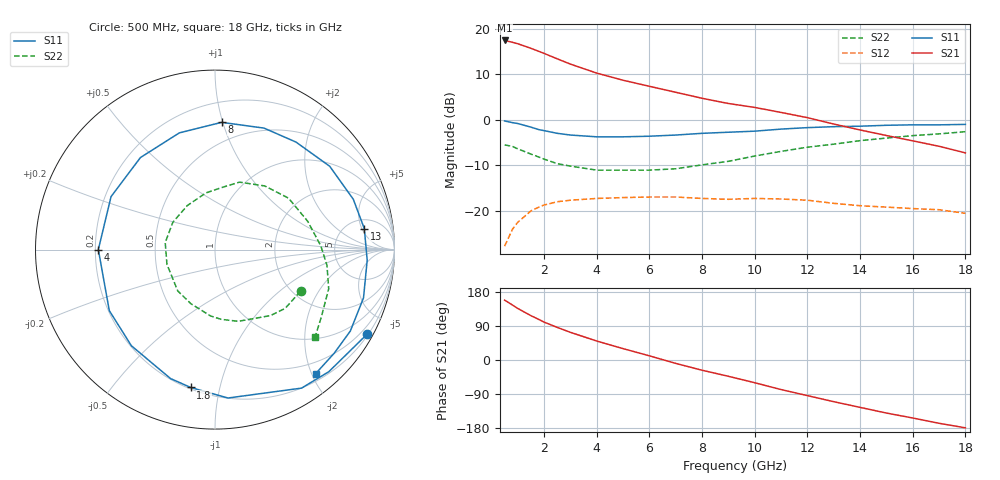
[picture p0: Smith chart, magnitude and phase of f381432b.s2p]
!ATF-38143
!S-PARAMETERS at Vds=2V  Id=10mA.  LAST UPDATED 20-10-99
# ghz s ma r 50
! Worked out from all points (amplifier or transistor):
!   23 points, 500 MHz to 18 GHz, reference 50 ohm
!   highest |S21| = 17.4 dB at 500 MHz (marker M1)
!   |S21| within 3 dB of that: start of sweep to 2.065 GHz
!   unconditionally stable (mu >= 1): 7.256 GHz to end of sweep
!   at 1.5 GHz: K = 0.27, MSG = 17.8 dB, |S12| = -20.0 dB
!   at 7 GHz: K = 0.97, MSG = 11.5 dB, |S12| = -17.0 dB
!   at 18 GHz: K = 1.55, MAG = 2.3 dB, |S12| = -20.5 dB
!   lowest NFmin = 0.18 dB at 500 MHz
!   S11 on the Smith chart (normalised r, x): 500 MHz: 0.24, -3.85; 1.8 GHz: 0.21, -0.82; 4 GHz: 0.21, +0.00; 8 GHz: 0.35, +0.99; 13 GHz: 7.02, +5.57; 18 GHz: 0.31, -2.06
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0.5  0.97 -29.0  7.423 158.0  0.041 72.0  0.53 -26.0
0.8  0.93 -47.0  7.081 145.0  0.063 61.0  0.51 -40.0
1  0.91 -58.0  6.834 136.0  0.075 55.0  0.48 -50.0
1.5  0.83 -85.0  6.086 117.0  0.1 40.0  0.42 -72.0
1.8  0.78 -100.0  5.634 107.0  0.11 33.0  0.39 -85.0
2  0.76 -109.0  5.35 100.0  0.116 28.0  0.37 -94.0
2.5  0.71 -131.0  4.665 86.0  0.126 18.0  0.33 -114.0
3  0.68 -150.0  4.083 73.0  0.131 9.0  0.31 -132.0
4  0.65 180.0  3.251 50.0  0.137 -5.0  0.28 -163.0
5  0.65 153.0  2.716 30.0  0.14 -18.0  0.28 172.0
6  0.66 129.0  2.33 11.0  0.142 -30.0  0.28 147.0
7  0.68 107.0  2.003 -9.0  0.142 -42.0  0.29 122.0
8  0.71 87.0  1.722 -27.0  0.137 -53.0  0.32 99.0
9  0.73 68.0  1.509 -43.0  0.134 -62.0  0.35 83.0
10  0.75 53.0  1.366 -60.0  0.137 -72.0  0.4 70.0
11  0.79 36.0  1.204 -78.0  0.135 -83.0  0.45 52.0
13  0.84 8.0  0.898 -110.0  0.121 -104.0  0.54 17.0
14  0.85 -4.0  0.773 -125.0  0.114 0.1  0.59 2.0
15  0.87 -18.0  0.672 -140.0  0.11 -122.0  0.63 -8.0
16  0.88 -31.0  0.587 -153.0  0.106 -131.0  0.67 -19.0
17  0.88 -41.0  0.512 -167.0  0.103 0.1  0.7 -32.0
18  0.89 -51.0  0.433 -179.0  0.094 -148.0  0.74 -41.0
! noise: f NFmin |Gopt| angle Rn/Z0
0.5  0.18  0.66  13  0.17
0.9  0.19  0.64  22  0.16
1.5  0.23  0.6  43  0.14
1.8  0.25  0.57  60  0.12
2.5  0.32  0.54  81  0.1
3  0.39  0.52  98  0.08
5  0.65  0.44  166  0.04
6  0.75  0.45  -165  0.04
8  0.95  0.51  -106  0.16
10  1.2  0.56  -65  0.46
